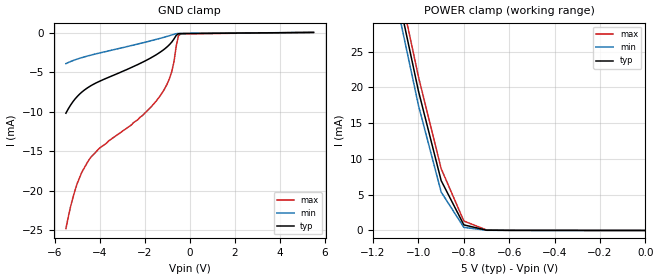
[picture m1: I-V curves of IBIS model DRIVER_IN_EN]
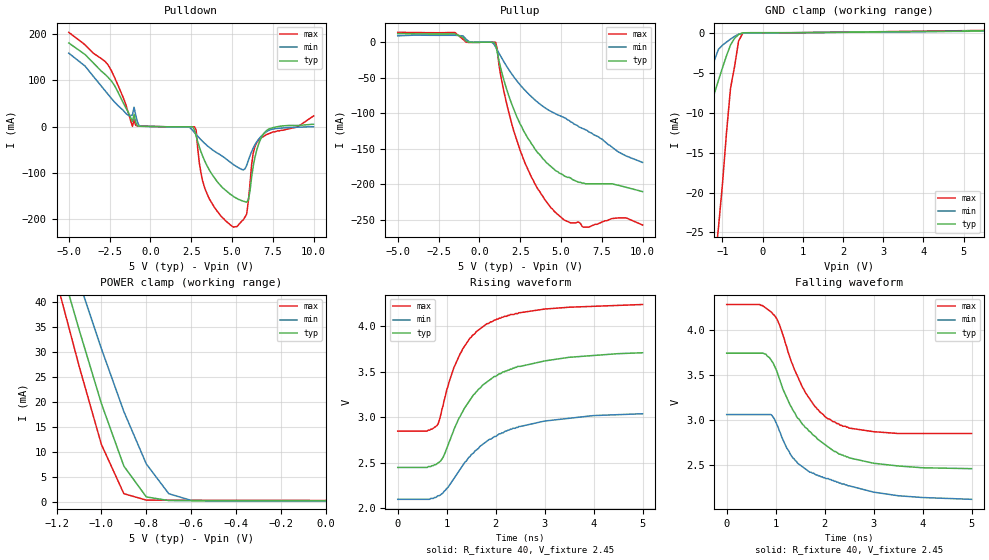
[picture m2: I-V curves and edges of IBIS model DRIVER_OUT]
|   Texas Instruments Incorporated
|   Data Transmissions Products
|   IBIS Model for TB5D1M
|   16DW SOIC Package
[IBIS Ver]   3.2
[Comment char]   |_char
[File name]   tb5d1mdw.ibs
[File Rev]   1.0
[Date]   20Jan04
[Source]   File originated at Texas Instruments Incorporated.
   Data Transmission Products Group. All data based on
   Simulation.
[Notes]
[Disclaimer]
(C) Copyright Texas Instruments Incorporated 2004
   All rights reserved
  Texas Instruments Incorporated hereby grants the user of this IBIS
model a non-exclusive, nontransferable license to use this IBIS model
under the following terms.  Before using this IBIS model, the user
should read this license.  If the user does not accept these terms,
the IBIS model should be returned to Texas Instruments within 30 days.
  The user is granted this license only to use the IBIS model and
is not granted rights to sell, load, rent, lease or license the IBIS
model in whole or in part, or in modified form to anyone other than
user.  User may modify the IBIS model to suit its specific applications
but rights to derivative works and such modifications shall belong to
Texas Instruments.
  This IBIS model is provided on an "AS IS" basis and Texas Instruments
makes absolutely no warranty with respect to the information contained
herein.  TEXAS INSTRUMENTS DISCLAIMS AND CUSTOMER WAIVES ALL WARRANTIES,
EXPRESS OR IMPLIED, INCLUDING WARRANTIES OF MERCHANTABILITY OR FITNESS
FOR A PARTICULAR PURPOSE. The entire risk as to quality and performance
is with the Customer. ACCORDINGLY, IN NO EVENT SHALL THE COMPANY BE LIABLE
FOR ANY DAMAGES, WHETHER IN CONTRACT OR TORT,INCLUDING ANY LOST PROFITS
OR OTHER INCIDENTAL, CONSEQUENTIAL, EXEMPLARY, OR PUNITIVE DAMAGES ARISING
OUT OF THE USE OR APPLICATION OF THE IBIS model provided in this package.
Further, Texas Instruments reserves the right to discontinue or make changes
without notice to any product herein to improve reliability, function, or
design. Texas Instruments does not convey any license under patent rights
or any other intellectual property rights, including those of third parties.
Contact Texas Instruments at ATTN:DATA TRANSMISSIONS
[Copyright]   Copyright 2004, Texas Instruments, All Rights Reserved
[Component]   TB5D1M
[Manufacturer]  Texas Instruments
[Package]
|   typ   min   max
R_pkg   0.046   0.034   0.057
L_pkg   4.858nH   3.987nH   6.214nH
C_pkg   0.715pF   0.502pF   1.046pF
[Pin]   signal_name   model_name   R_pin   L_pin   C_pin
1   AI   DRIVER_IN_EN   0.057   6.214nH   1.026pF
2   AO   DRIVER_OUT   0.055   5.236nH   0.818pF
3   AO(-)   DRIVER_OUT   0.034   3.987nH   0.723pF
4   E1   DRIVER_IN_EN   0.036   3.996nH   0.726pF
5   BO(-)   DRIVER_OUT   0.036   3.996nH   0.726pF
6   BO   DRIVER_OUT   0.034   3.987nH   0.704pF
7   BI   DRIVER_IN_EN   0.055   5.236nH   0.818pF
8   GND   GND   0.057   6.214nH   1.046pF
9   CI   DRIVER_IN_EN   0.057   6.214nH   0.827pF
10   CO   DRIVER_OUT   0.055   5.236nH   0.597pF
11   CO(-)   DRIVER_OUT   0.034   3.987nH   0.502pF
12   E2   DRIVER_IN_EN   0.036   3.996nH   0.505pF
13   DO(-)   DRIVER_OUT   0.036   3.996nH   0.505pF
14   DO   DRIVER_OUT   0.034   3.987nH   0.502pF
15   DI   DRIVER_IN_EN   0.055   5.236nH   0.597pF
16   VCC   POWER   0.057   6.214nH   0.827pF
[Diff_pin]   inv_pin   vdiff   tdelay_typ   tdelay_min   tdelay_max
| The 'AO(+) (or 'xO(+)')' and inv_pins, 'AO(-) (or 'xO(-)')', pins
| are Diff_pins
   2   3   0   0   0   0
   6   5   0   0   0   0
   10   11   0   0   0   0
   14   13   0   0   0   0
| Models and submodels in the file (2): DRIVER_IN_EN (Input), DRIVER_OUT (Output_ECL)
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|   Driver Input Model
[Model]   DRIVER_IN_EN
Model_type   Input
|Signals   AI,BI,CI,DI,E1,E2
Vinh = 2.4
Vinl = 0.4
|   typ   min   max
C_comp   964fF   924fF   1010fF
|   typ   min   max
[Temperature Range]   25.0   -40.0   125.0
[Voltage range]   5.0V   4.5V   5.5V
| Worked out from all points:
|   GND clamp passes 1 mA (typ) near -0.75 V on its own axis
|   POWER clamp passes 1 mA (typ) near -0.80 V on its own axis
[GND_clamp]
| Voltage   I(typ)   I(min)   I(max)
-5.5V     -10.2mA    -3.93mA    -24.8mA
-5.3V     -9.21mA    -3.68mA    -22.1mA
-5V       -8.1mA     -3.36mA    -19.1mA
-4.5V     -6.92mA    -2.94mA    -16.2mA
-4V       -6.16mA    -2.59mA    -14.6mA
-2.1V     -3.76mA    -1.31mA    -10.5mA
-1.5V     -2.83mA    -876uA     -8.7mA
-1.1V     -2.04mA    -566uA     -7.04mA
-800mV    -1.21mA    -311uA     -4.96mA
-700mV    -818uA     -220uA     -3.71mA
-500mV    -158uA     -114uA     -389uA
5.5V      13.6uA     12uA       16.5uA
[Power_clamp]
| Note that the[POWER_clamp]voltage table is referenced to Vcc
| and is calculated using Vtable=Vcc - Vmeasured.
|   Voltage   I(typ)   I(min)   I(max)
-5V       324mA      323mA      330mA
-1.1V     34.4mA     32.4mA     36.4mA
-1V       19.5mA     17.5mA     21.5mA
-900mV    6.98mA     5.38mA     8.65mA
-800mV    782uA      431uA      1.32mA
-700mV    41.2uA     26.6uA     71.3uA
0V        1.02uA     1.75uA     633nA
|   Driver Output Model
[Model]   DRIVER_OUT
|Model_type   3-state_ECL
Model_type   Output_ECL
| Signals   O(+),O(-)
Vmeas = 3.2V   |Reference voltage for timing measurements
Cref = 0pF   |Timing specification test load capacitance value
Rref = 40   |Note: 40 Ohm load; single ended configuration
| variable   typ   min   max
C_comp   970fF   930fF   1010fF
|   typ   min   max
[Temperature Range]   25.0   -40.0   125.0
[Voltage range]   5.0V   4.5V   5.5V
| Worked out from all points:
|   GND clamp passes 1 mA (typ) near -0.74 V on its own axis
|   POWER clamp passes 1 mA (typ) near -0.80 V on its own axis
|   rising waveform, R_fixture 40, V_fixture 2.45: 20-80 % time 987ps typ, 1.13ns min, 731ps max; typ from 2.45 V to 3.71 V
|   falling waveform, R_fixture 40, V_fixture 2.45: 20-80 % time 975ps typ, 1.2ns min, 714ps max; typ from 3.74 V to 2.46 V
[Pulldown]
|Voltage I(typ)   I(min)   I(max)
-5V       181mA      159mA      204mA
-2.6V     107mA      70.3mA     134mA
-1.1V     11.5mA     25.3mA     830uA
2.7V      -7.28mA    -12.5mA    -119uA
3.4V      -79.3mA    -38.3mA    -139mA
5.1V      -151mA     -82mA      -217mA
5.9V      -163mA     -83.4mA    -189mA
6V        -158mA     -73.1mA    -161mA
6.3V      -85.6mA    -46.1mA    -57.3mA
6.6V      -40.9mA    -28.4mA    -30.2mA
7.3V      -4.43mA    -7.11mA    -14.4mA
10V       5.42mA     36.8uA     23.4mA
[Pullup]
|   Voltage   I(typ)   I(min)   I(max)
| Note that the[Pullup]voltage table is referenced to Vcc
| and is calculated using Vtable=Vcc - Vmeasured.
-5V       12.1mA     8.97mA     13.9mA
-1.5V     11.7mA     9.75mA     13.7mA
-1V       6.79mA     8.88mA     4.07mA
1V        -3.83mA    -6.8mA     -208uA
1.6V      -60.7mA    -31.1mA    -79mA
2.5V      -115mA     -60mA      -152mA
3.4V      -150mA     -81mA      -199mA
4.4V      -175mA     -97.4mA    -233mA
5.2V      -188mA     -106mA     -250mA
6.4V      -198mA     -122mA     -260mA
8.5V      -201mA     -154mA     -247mA
10V       -210mA     -169mA     -257mA
[GND_clamp]
|   Voltage   I(typ)   I(min)   I(max)
| Outputs in High Impedance (off)
-5.5V     -216mA     -169mA     -280mA
-1.6V     -38.7mA    -41.9mA    -110mA
-1.5V     -18.9mA    -29.8mA    -72.8mA
-1.4V     -11.8mA    -17.5mA    -44.1mA
-1.3V     -9.26mA    -7.94mA    -36.7mA
-1.2V     -7.56mA    -3.42mA    -29.3mA
-1.1V     -5.96mA    -2.07mA    -24.4mA
-800mV    -1.53mA    -797uA     -6.95mA
-600mV    -217uA     -186uA     -1.06mA
-500mV    -20.4uA    -56.3uA    -92.9uA
-400mV    -1.07uA    -12.6uA    -4.4uA
5.5V      232uA      201uA      288uA
[Power_clamp]
| Note that the[POWER_clamp]voltage table is referenced to Vcc
| and is calculated using Vtable=Vcc - Vmeasured.
|Voltage  I(typ)   I(min)   I(max)
-5V       327mA      316mA      338mA
-1.2V     50.2mA     58.1mA     44.3mA
-1.1V     34.6mA     44.2mA     27.3mA
-1V       19.7mA     30.7mA     11.5mA
-900mV    7.17mA     18.1mA     1.64mA
-800mV    998uA      7.61mA     351uA
-700mV    264uA      1.64mA     328uA
-600mV    237uA      296uA      322uA
0V        207uA      154uA      285uA
[Ramp]
|   typ   min   max
dV/dt_r   0.774/1069ps   0.577/1207ps   0.858/804ps
dV/dt_f   0.774/979ps   0.575/1271ps   0.859/707ps
R_load = 40ohm
[Rising Waveform]
R_fixture = 40
V_fixture = 2.45
V_fixture_min = 2.05
V_fixture_max = 2.85
C_fixture = 0
|   V(typ)  V(min)  V(max)
0s        2.45V      2.1V       2.85V
800ps     2.49V      2.13V      2.91V
925ps     2.56V      2.17V      3.13V
1.05ns    2.73V      2.25V      3.39V
1.275ns   3.01V      2.43V      3.7V
1.475ns   3.19V      2.57V      3.87V
1.825ns   3.39V      2.74V      4.03V
2.45ns    3.56V      2.89V      4.14V
3ns       3.62V      2.96V      4.19V
5ns       3.71V      3.04V      4.24V
[Falling Waveform]
R_fixture = 40
V_fixture = 2.45
V_fixture_min = 2.05
V_fixture_max = 2.85
C_fixture = 0
|   V(typ)  V(min)  V(max)
0s        3.74V      3.06V      4.28V
750ps     3.74V      3.06V      4.26V
925ps     3.65V      3.05V      4.19V
1.075ns   3.46V      2.88V      4.06V
1.225ns   3.25V      2.69V      3.81V
1.45ns    3.02V      2.52V      3.48V
1.8ns     2.82V      2.4V       3.15V
2.175ns   2.66V      2.33V      2.98V
3ns       2.52V      2.2V       2.87V
5ns       2.46V      2.12V      2.85V
